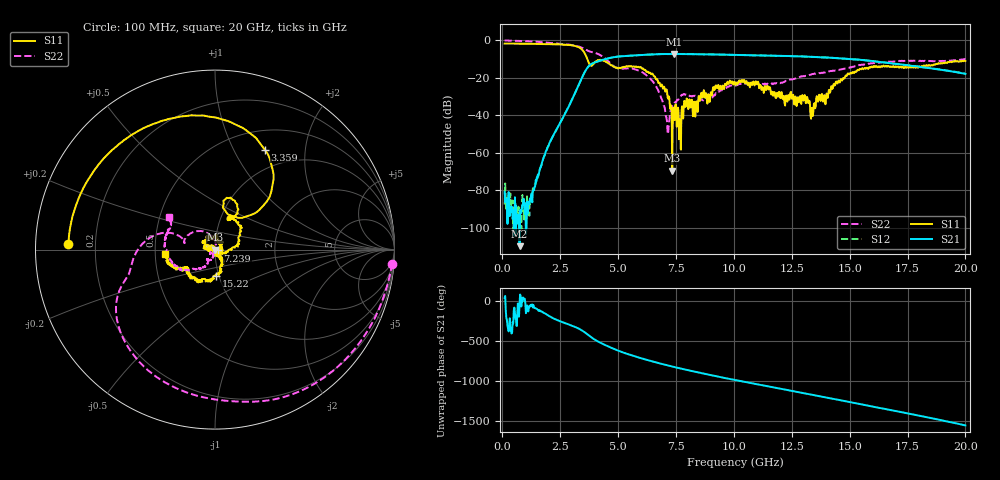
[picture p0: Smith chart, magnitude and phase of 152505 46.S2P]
!  2-Port S-parameters saved by WinCal
! VAR MeasName=S-Parameters (CALIBRATED_DATA) read from VNA (N5230C)
! VAR MeasDate=4/10/2015 9:33:07 AM
! VAR NAME=152505 46
! VAR FILENAME=152505 46.S2P
! VAR DATE=4/10/2015 9:33:07 AM
! VAR PHYS_PORTS=1,2
# Hz S DB R 50
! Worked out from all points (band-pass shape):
!   801 points, 100 MHz to 20 GHz, reference 50 ohm
!   highest |S21| = -7.29 dB at 7.413 GHz (marker M1); lowest = -109.8 dB at 746.8 MHz (marker M2)
!   |S21| within 3 dB of the highest: 4.373 GHz to 15.36 GHz (10.98 GHz wide, 111 % of centre)
!   lowest |S11| = -69.6 dB at 7.339 GHz (marker M3), VSWR 1.00, Z = 50 - j0.0331 ohm
!   |S11| at or under -10 dB: 3.671 GHz to end of sweep
!   |S22| runs from -50.0 to -0.1 dB; largest |S21 - S12| = 0.0054
!   S11 on the Smith chart (normalised r, x): 100 MHz: 0.10, +0.02; 3.359 GHz: 0.74, +1.34; 7.239 GHz: 1.03, -0.01; 15.22 GHz: 0.97, -0.29; 20 GHz: 0.56, -0.03
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1e8  -1.75 177.6  -80.87 38.2  -87.63 76.9  -0.09 -4.6
7.4675e8  -1.80 162.2  -109.83 -18.5  -91.30 45.7  -0.35 -30.3
1.318875e9  -1.89 147.9  -80.20 -81.3  -79.00 -76.0  -0.63 -53.5
2.413375e9  -2.17 115.5  -45.93 115.3  -45.98 114.9  -1.75 -98.1
3.358625e9  -4.12 63.5  -22.18 4.7  -22.18 5.1  -3.57 -145.9
3.43325e9  -4.84 57.0  -20.15 -7.9  -20.14 -7.7  -3.93 -150.2
3.83125e9  -13.56 64.6  -12.76 -93.3  -12.79 -93.2  -6.17 -165.5
4.403375e9  -11.00 64.0  -10.18 172.8  -10.20 172.8  -9.33 166.1
5.1745e9  -14.37 68.2  -8.50 78.7  -8.53 78.8  -15.17 167.7
5.945625e9  -14.41 39.0  -7.93 6.3  -7.91 6.4  -16.37 139.2
6.741625e9  -22.76 -3.9  -7.40 -58.1  -7.40 -58.2  -27.07 88.9
7.11475e9  -27.38 -17.9  -7.33 -86.2  -7.33 -86.0  -43.28 25.2
7.239125e9  -35.39 -16.8  -7.31 -95.0  -7.29 -94.9  -39.97 -99.0
7.338625e9  -69.56 -94.5  -7.30 -102.2  -7.28 -102.2  -34.79 -112.4
7.41325e9  -39.36 -84.6  -7.29 -107.2  -7.30 -107.3  -33.88 -112.3
8.582375e9  -28.28 145.3  -7.44 175.9  -7.41 175.8  -31.66 -140.9
1.005e10  -22.42 141.7  -7.76 88.8  -7.80 88.7  -24.06 -114.2
1.169175e10  -29.48 36.3  -8.23 -2.2  -8.23 -2.5  -23.40 -124.5
1.338325e10  -36.09 -95.6  -8.86 -96.1  -8.83 -95.9  -17.99 -125.1
1.5224e10  -16.78 -88.2  -10.23 159.9  -10.18 159.9  -13.80 -145.9
1.669162e10  -13.81 -133.6  -12.12 76.2  -12.06 75.5  -11.44 -174.1
2e10  -11.05 -174.8  -17.88 -121.4  -17.87 -121.3  -10.03 144.8
